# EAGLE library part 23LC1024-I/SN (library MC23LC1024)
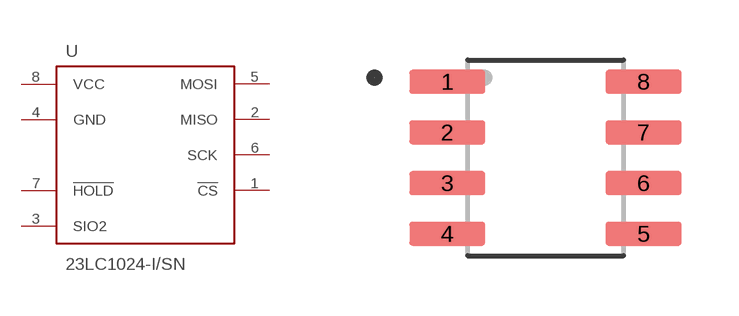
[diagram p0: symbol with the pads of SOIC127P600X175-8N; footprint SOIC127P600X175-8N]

Designator prefix -

## 23LC1024-I/SN  [SOIC127P600X175-8N]
1  !CS!
2  MISO
3  SIO2
4  GND
5  MOSI
6  SCK
7  !HOLD!
8  VCC

## Footprint SOIC127P600X175-8N (pad centres in mm)
smd 1.9 x 0.6: 1 -2.455,1.905; 2 -2.455,0.635; 3 -2.455,-0.635; 4 -2.455,-1.905; 5 2.455,-1.905; 6 2.455,-0.635; 7 2.455,0.635; 8 2.455,1.905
